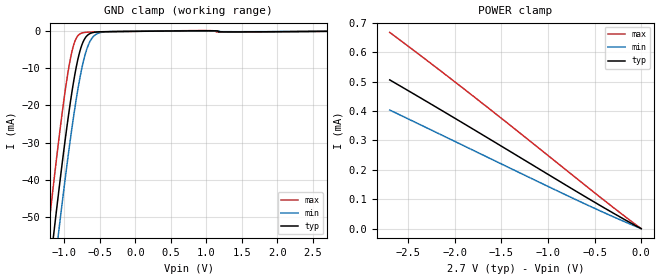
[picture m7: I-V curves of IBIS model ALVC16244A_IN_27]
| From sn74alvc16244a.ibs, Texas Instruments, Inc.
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[Model]   ALVC16244A_IN_27
Model_type  Input
Vinl=0.7
Vinh=1.7
| variable   typ   min   max
C_comp   0.96pF   0.64pF   1.19pF
[Temperature Range]   40   100   -40
| Ambient temperature   25   85   -40
[Voltage range]   2.7   2.7   2.7
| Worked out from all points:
|   GND clamp passes 1 mA (typ) near -0.67 V on its own axis
[GND Clamp]
| ALVC16244A_IN_27
|   Voltage   I(typ)   I(min)   I(max)
-2.7V     -338.2mA   -347.4mA   -327.1mA
-1.24V    -69.59mA   -80.37mA   -55.77mA
-1.16V    -56.1mA    -66.91mA   -42.2mA
-1.135V   -51.97mA   -62.78mA   -38.08mA
-1.075V   -42.29mA   -53.04mA   -28.49mA
-985mV    -28.56mA   -39.05mA   -15.41mA
-910mV    -18.28mA   -28.19mA   -6.803mA
-850mV    -11.28mA   -20.29mA   -2.557mA
-775mV    -4.878mA   -11.87mA   -624.8uA
-650mV    -710.4uA   -3.103mA   -211.8uA
-485mV    -123.2uA   -304.6uA   -147.3uA
2.7V      1.115nA    59.61nA    7.183pA
[POWER Clamp]
| ALVC16244A_IN_27
|   Voltage   I(typ)   I(min)   I(max)
-2.7V     505.5uA    403.1uA    666.9uA
-1.815V   340.1uA    268uA      453.1uA
-735mV    134uA      103.6uA    181.2uA
-35.59fV  1.115nA    59.61nA    7.183pA
